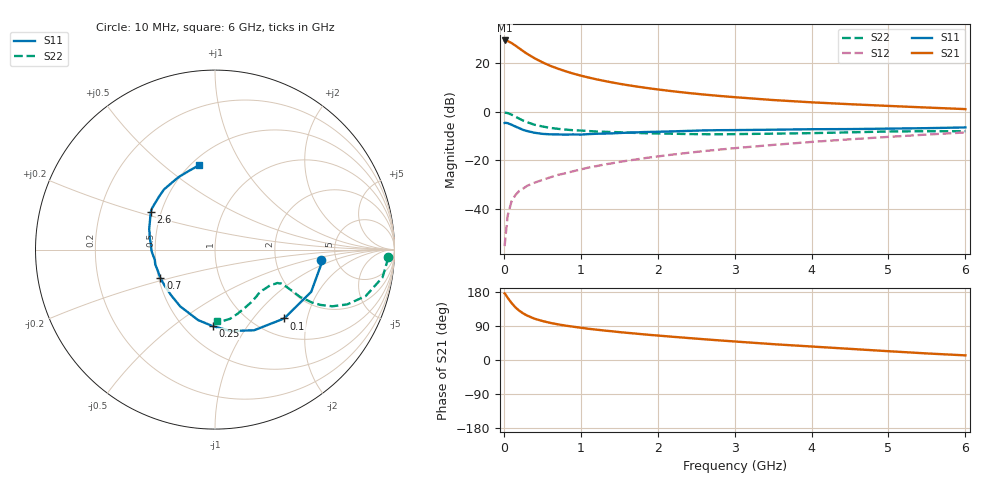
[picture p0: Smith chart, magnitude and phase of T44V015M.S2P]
! Infineon Technologies  Discrete & RF Semiconductors
! BFR182T
! Si NPN RF Bipolar Junction Transistor in SC75
! VCE = 4 V  IC = 15 mA
! Common Emitter S-Parameters:  October  1999
# GHz  S  MA  R  50
!  f  S11  S21  S12  S22
! GHz  MAG  ANG  MAG  ANG  MAG  ANG  MAG  ANG
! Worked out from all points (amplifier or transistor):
!   36 points, 10 MHz to 6 GHz, reference 50 ohm
!   highest |S21| = 29.5 dB at 10 MHz (marker M1)
!   |S21| within 3 dB of that: start of sweep to 189.2 MHz
!   unconditionally stable (mu >= 1): 789.5 MHz to 3.707 GHz
!   at 250 MHz: K = 0.56, MSG = 28.4 dB, |S12| = -31.7 dB
!   at 1.4 GHz: K = 1.09, MAG = 14.9 dB, |S12| = -21.2 dB
!   at 6 GHz: K = 0.85, MSG = 4.8 dB, |S12| = -8.5 dB
!   S11 on the Smith chart (normalised r, x): 10 MHz: 3.76, -0.69; 100 MHz: 1.34, -1.46; 250 MHz: 0.68, -0.71; 700 MHz: 0.51, -0.18; 2.6 GHz: 0.44, +0.22; 6 GHz: 0.55, +0.67
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0.01  0.5912 -5.8  29.77 175.6  0.0017 84.0  0.9643 -2.6
0.02  0.5966 -8.2  29.64 173.7  0.0025 100.8  0.9626 -3.7
0.05  0.5854 -23.7  28.89 164.2  0.0073 80.8  0.946 -9.4
0.1  0.5437 -44.9  26.37 150.5  0.0143 74.4  0.8791 -17.1
0.15  0.4996 -64.1  23.34 139.0  0.0192 66.9  0.7976 -22.5
0.2  0.4619 -79.1  20.49 130.1  0.0234 65.5  0.7259 -25.8
0.25  0.4262 -91.8  17.96 123.2  0.0261 61.6  0.6626 -27.7
0.3  0.404 -103.4  15.88 117.5  0.0297 61.6  0.6155 -28.6
0.4  0.3711 -121.5  12.76 108.9  0.0347 61.4  0.5427 -29.1
0.5  0.3526 -134.1  10.57 103.0  0.0394 62.6  0.5009 -28.4
0.6  0.345 -144.7  8.979 98.1  0.0445 64.1  0.4698 -27.9
0.7  0.3431 -152.5  7.825 94.2  0.05 65.5  0.4477 -27.5
0.9  0.343 -166.0  6.182 87.9  0.0596 67.5  0.4189 -27.2
1.1  0.3479 -175.6  5.124 82.4  0.071 68.1  0.4033 -27.8
1.3  0.3568 176.7  4.377 77.9  0.0819 68.7  0.3894 -28.9
1.6  0.3727 167.8  3.585 71.8  0.0982 69.1  0.3741 -31.0
2.2  0.397 155.8  2.659 61.2  0.1321 68.7  0.3548 -37.7
2.6  0.4152 149.4  2.283 54.8  0.1554 67.8  0.3471 -42.8
3.5  0.4293 136.6  1.757 41.8  0.2084 64.7  0.356 -55.5
4.5  0.4422 124.2  1.441 29.4  0.2721 59.7  0.3787 -70.5
5.5  0.4621 108.3  1.23 17.3  0.3408 53.8  0.3997 -83.4
6  0.4783 100.6  1.142 12.2  0.3769 50.2  0.3997 -88.6
